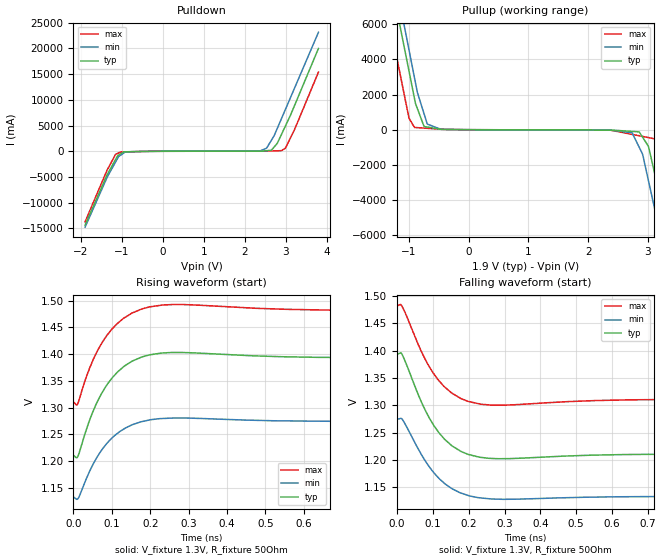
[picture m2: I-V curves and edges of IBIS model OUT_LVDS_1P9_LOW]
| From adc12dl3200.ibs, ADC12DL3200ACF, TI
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|   OUT_LVDS_1P9_LOW
[Model]   OUT_LVDS_1P9_LOW
Model_type   Output
Polarity   Non-Inverting
Vmeas = 1.3
Vref = 1.3
Cref = 2pF
Rref = 50
|   typ   min   max
C_comp   1.666E-12   1.540E-12   1.713E-12
[Voltage Range]   1.9   1.8   2
[Temperature Range]   90   150   -55
[Pullup Reference]   1.9   1.8   2
[Pulldown Reference]   -0   0   -0
[Power Clamp Reference]   1.9   1.8   2
[GND Clamp Reference]   0   0   0
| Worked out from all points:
|   slope of the pulldown table from 0 to 0.285 V, typ, clamps not added: 63.1 ohm
|   slope of the pullup table from 0 to 0.285 V, typ, clamps not added: 78.3 ohm
|   falling waveform, V_fixture 1.3V, R_fixture 50Ohm: 20-80 % time 83.5ps typ, 86.8ps min, 80.5ps max; typ from 1.39 V to 1.21 V
|   rising waveform, V_fixture 1.3V, R_fixture 50Ohm: 20-80 % time 74ps typ, 74.4ps min, 73.7ps max; typ from 1.21 V to 1.39 V
[Pulldown]
|   Voltage   I(typ)   I(min)   I(max)
-1.9V     -14.37A    -14.78A    -13.74A
-1.362V   -4.602A    -5.096A    -3.689A
-1.156V   -1.621A    -2.114A    -631.9mA
-1.079V   -746.2mA   -1.025A    -325.1mA
-915.9mV  -112.4mA   -125.2mA   -125.7mA
2.322V    15.59mA    23.53mA    11.29mA
2.535V    106.7mA    605mA      39.54mA
2.651V    191.8mA    2.15A      61.88mA
2.794V    1.537A     4.431A     89.19mA
2.995V    4.942A     8.176A     613.8mA
3.224V    9.048A     12.43A     4.365A
3.8V      20A        23.14A     15.39A
[Pullup]
|   Voltage   I(typ)   I(min)   I(max)
-1.9V     20A        21.21A     17.34A
-1.258V   7.793A     9.033A     4.994A
-1.002V   3.363A     4.564A     690.9mA
-907.5mV  1.765A     2.945A     130.1mA
-693.3mV  152.7mA    320.4mA    81.46mA
-463.9mV  23.89mA    24.37mA    29.36mA
2.737V    -94.91mA   -170.5mA   -264mA
3.009V    -929.6mA   -2.849A    -443.4mA
3.146V    -2.917A    -4.95A     -534mA
3.234V    -4.219A    -6.309A    -1.798A
3.352V    -6.213A    -8.468A    -3.513A
3.8V      -14.37A    -16.65A    -11.82A
[Ramp]
R_load = 50
|   typ   min   max
dV/dt_r   0.109677/7.40833e-11  0.0847789/7.45248e-11   0.10253/7.37741e-11
dV/dt_f   0.109666/8.34488e-11  0.0847655/8.67631e-11   0.10252/8.03954e-11
[Falling Waveform]
V_fixture = 1.3V
V_fixture_min = 1.2V
V_fixture_max = 1.4V
R_fixture = 50Ohm
C_fixture = 0F
|   Time   V(typ)   V(min)   V(max)
0s        1.393V     1.274V     1.482V
9.74ps    1.396V     1.276V     1.485V
13.86ps   1.393V     1.275V     1.481V
81.17ps   1.288V     1.196V     1.381V
101.9ps   1.264V     1.177V     1.358V
132.7ps   1.238V     1.157V     1.334V
178.9ps   1.215V     1.139V     1.312V
256.4ps   1.203V     1.129V     1.301V
769.9ps   1.211V     1.133V     1.311V
5ns       1.211V     1.133V     1.311V
[Rising Waveform]
V_fixture = 1.3V
V_fixture_min = 1.2V
V_fixture_max = 1.4V
R_fixture = 50Ohm
C_fixture = 0F
|   Time   V(typ)   V(min)   V(max)
0s        1.211V     1.133V     1.311V
10.87ps   1.208V     1.129V     1.306V
35ps      1.262V     1.169V     1.36V
60.03ps   1.308V     1.206V     1.403V
90.52ps   1.346V     1.236V     1.438V
115.9ps   1.367V     1.253V     1.458V
178.9ps   1.395V     1.274V     1.485V
256.4ps   1.403V     1.28V      1.493V
769.9ps   1.393V     1.274V     1.482V
5ns       1.393V     1.274V     1.482V
